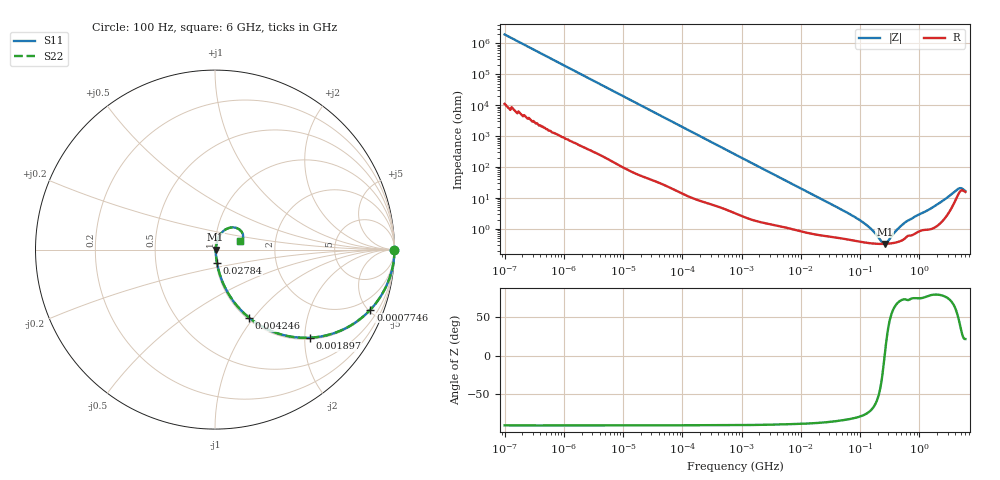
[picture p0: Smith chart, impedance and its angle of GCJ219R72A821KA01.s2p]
!Murata Part Number: GCJ219R72A821KA01
!These Parameters are Measured in Series Mode Connection
!Data Generated on Mar 13, 2026
!  o--ll--o
!Port1  Port2
!  o------o
!Operation Temp=25[degC], DC Bias Voltage=0[V]
!Freq. Start=100[Hz] Stop=6[GHz] 401[Steps]
# Hz S RI R 50
!Freq.(Hz) S11(Real) S11(Imag) S21(Real) S21(Imag) S12(Real) S12(Imag) S22(Real) S22(Imag)
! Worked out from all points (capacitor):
!   401 points, 100 Hz to 6 GHz, reference 50 ohm
!   read as one part in series: C = 824 pF near 109 Hz
!   lowest |Z| = 330 mohm at 261.2 MHz (marker M1)
!   series resonance near 260.5 MHz, so ESL is about 450 pH
!   S11 on the Smith chart (normalised r, x): 100 Hz: open; 774.6 kHz: 1.06, -5.15; 1.897 MHz: 1.03, -2.11; 4.246 MHz: 1.02, -0.95; 27.84 MHz: 1.01, -0.15; 6 GHz: 1.31, +0.12
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100  1 -5.19e-05  3e-07 5.19e-05  3e-07 5.19e-05  1 -5.19e-05
205  1 -0.000106  5e-07 0.000106  5e-07 0.000106  1 -0.000106
2008  1 -0.00103  6.1e-06 0.00103  6.1e-06 0.00103  1 -0.00103
40335  0.9994 -0.0205  0.000553 0.0205  0.000553 0.0205  0.9994 -0.0205
221108  0.9867 -0.1103  0.0133 0.1103  0.0133 0.1103  0.9867 -0.1103
774597  0.8657 -0.3348  0.1343 0.3348  0.1343 0.3348  0.8657 -0.3348
1896632  0.5269 -0.4911  0.4731 0.4911  0.4731 0.4911  0.5269 -0.4911
4246196  0.1904 -0.3797  0.8096 0.3797  0.8096 0.3797  0.1904 -0.3797
7266822  0.0802 -0.2546  0.9198 0.2546  0.9198 0.2546  0.0802 -0.2546
1.555665e7  0.0236 -0.1277  0.9764 0.1277  0.9764 0.1277  0.0236 -0.1277
2.784235e7  0.0111 -0.0726  0.9889 0.0726  0.9889 0.0726  0.0111 -0.0726
1.115611e8  0.00398 -0.0159  0.996 0.0159  0.996 0.0159  0.00398 -0.0159
1.596157e8  0.00347 -0.00863  0.9965 0.00863  0.9965 0.00863  0.00347 -0.00863
2.388273e8  0.00328 -0.00148  0.9967 0.00148  0.9967 0.00148  0.00328 -0.00148
2.61201e8  0.00329 5.01e-05  0.9967 -5.01e-05  0.9967 -5.01e-05  0.00329 5.01e-05
3.124326e8  0.00338 0.00315  0.9966 -0.00315  0.9966 -0.00315  0.00338 0.00315
4.274388e8  0.00383 0.00895  0.9962 -0.00895  0.9962 -0.00895  0.00383 0.00895
6.11557e8  0.00582 0.0166  0.9942 -0.0166  0.9942 -0.0166  0.00582 0.0166
2.562649e9  0.0256 0.0788  0.9744 -0.0788  0.9744 -0.0788  0.0256 0.0788
4.385646e9  0.119 0.1207  0.881 -0.1207  0.881 -0.1207  0.119 0.1207
5.016141e9  0.1554 0.0858  0.8446 -0.0858  0.8446 -0.0858  0.1554 0.0858
6e9  0.1377 0.0453  0.8623 -0.0453  0.8623 -0.0453  0.1377 0.0453
